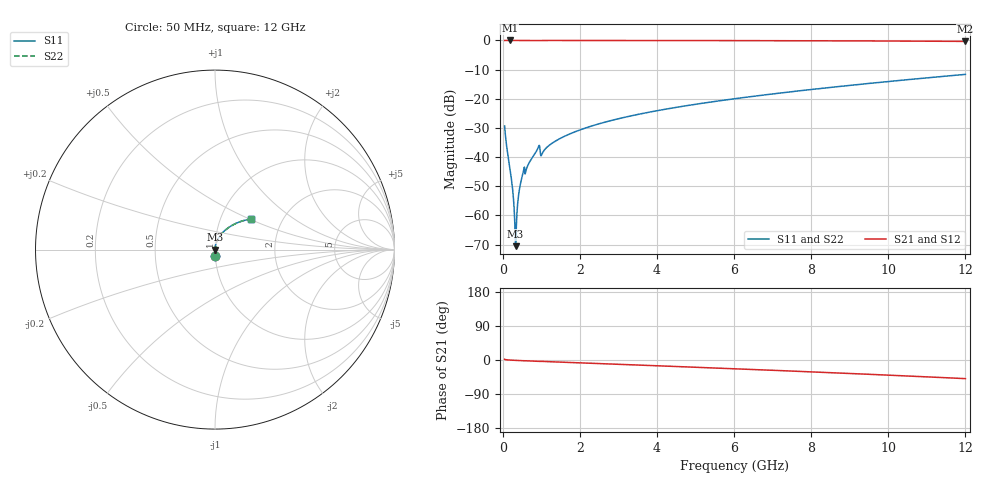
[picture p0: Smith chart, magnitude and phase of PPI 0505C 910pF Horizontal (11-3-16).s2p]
# MHz S MA R 50
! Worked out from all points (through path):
!   1601 points, 50 MHz to 12 GHz, reference 50 ohm
!   highest |S21| = 0.00 dB at 184.4 MHz (marker M1); lowest = -0.3 dB at 12 GHz (marker M2)
!   group delay of S21, straight-line fit = 11.3 ps
!   lowest |S11| = -70.5 dB at 333.8 MHz (marker M3), VSWR 1.00, Z = 50 - j0.00525 ohm
!   |S11| at or under -10 dB: start of sweep to end of sweep
!   |S22| runs from -70.5 to -11.6 dB; largest |S21 - S12| = 0
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50  0.03415 -87.9  0.9992 1.8  0.9992 1.8  0.03415 -87.9
87.34375  0.01865 -88.6  0.9996 0.8  0.9996 0.8  0.01865 -88.6
184.4375  0.006627 -88.0  0.9997 -0.2  0.9997 -0.2  0.006627 -88.0
244.1875  0.003387 -86.0  0.9997 -0.5  0.9997 -0.5  0.003387 -86.0
296.4688  0.001327 -78.5  0.9997 -0.8  0.9997 -0.8  0.001327 -78.5
333.8125  0.000298 -10.1  0.9997 -1.0  0.9997 -1.0  0.000298 -10.1
371.1562  0.001117 73.0  0.9997 -1.1  0.9997 -1.1  0.001117 73.0
386.0938  0.001529 77.1  0.9997 -1.2  0.9997 -1.2  0.001529 77.1
415.9688  0.002332 80.8  0.9997 -1.3  0.9997 -1.3  0.002332 80.8
438.375  0.002917 82.1  0.9996 -1.4  0.9996 -1.4  0.002917 82.1
513.0625  0.004877 83.6  0.9996 -1.8  0.9996 -1.8  0.004877 83.6
901.4375  0.01362 81.8  0.9987 -3.4  0.9987 -3.4  0.01362 81.8
1035.875  0.01189 80.5  0.9987 -3.7  0.9987 -3.7  0.01189 80.5
1162.844  0.01509 83.5  0.9992 -4.3  0.9992 -4.3  0.01509 83.5
1371.969  0.0189 83.3  0.9992 -5.1  0.9992 -5.1  0.0189 83.3
2044.156  0.02993 81.3  0.9989 -7.7  0.9989 -7.7  0.02993 81.3
2910.531  0.04402 78.2  0.9982 -11.0  0.9982 -11.0  0.04402 78.2
4038.312  0.06313 74.0  0.997 -15.4  0.997 -15.4  0.06313 74.0
6025  0.1005 66.3  0.9937 -23.2  0.9937 -23.2  0.1005 66.3
8019.156  0.1448 58.2  0.988 -31.4  0.988 -31.4  0.1448 58.2
10013.31  0.1981 49.7  0.9784 -40.0  0.9784 -40.0  0.1981 49.7
12000  0.2621 40.5  0.9629 -49.2  0.9629 -49.2  0.2621 40.5
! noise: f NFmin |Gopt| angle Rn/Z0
50  0.0002962  0.8256  0.1822  0.0003569
1372  0.002756  0.5606  3.82  0.001126
2701  0.004295  0.4759  7.201  0.001388
4031  0.00574  0.4336  10.38  0.001661
5360  0.007117  0.4067  13.35  0.001921
6682  0.008466  0.3896  16.12  0.002184
8012  0.009838  0.3797  18.75  0.002466
9341  0.01126  0.3758  21.25  0.002779
1.067e+04  0.01275  0.3771  23.66  0.003137
1.2e+04  0.01435  0.3832  26.04  0.003554
